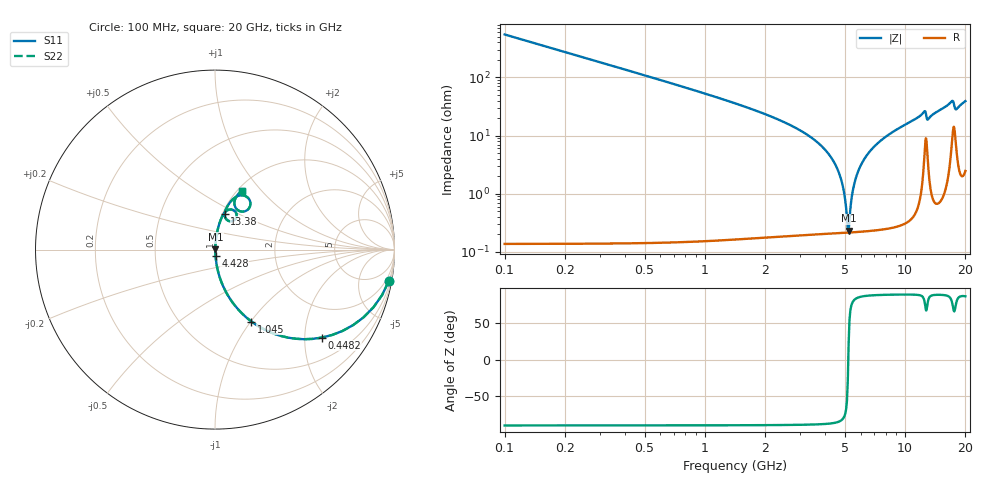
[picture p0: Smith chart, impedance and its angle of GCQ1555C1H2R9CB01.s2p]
!Murata Part Number: GCQ1555C1H2R9CB01
!These Parameters are Measured in Series Mode Connection
!Data Generated on Jan 08, 2026
!  o--ll--o
!Port1  Port2
!  o------o
!Operation Temp=25[degC], DC Bias Voltage=0[V]
!Freq. Start=100[MHz] Stop=20[GHz] 401[Steps]
# Hz S RI R 50
!Freq.(Hz) S11(Real) S11(Imag) S21(Real) S21(Imag) S12(Real) S12(Imag) S22(Real) S22(Imag)
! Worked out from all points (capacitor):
!   401 points, 100 MHz to 20 GHz, reference 50 ohm
!   read as one part in series: C = 2.9 pF near 199.5 MHz
!   lowest |Z| = 232 mohm at 5.224 GHz (marker M1)
!   series resonance near 5.203 GHz, so ESL is about 320 pH
!   S11 on the Smith chart (normalised r, x): 100 MHz: 1, -11; 448.2 MHz: 1.00, -2.43; 1.045 GHz: 1.00, -1.01; 4.428 GHz: 1.00, -0.07; 13.38 GHz: 1.02, +0.42; 20 GHz: 1.05, +0.78
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1e8  0.9678 -0.1764  0.0322 0.1764  0.0322 0.1764  0.9678 -0.1764
4.4825e8  0.5961 -0.4901  0.4039 0.4901  0.4039 0.4901  0.5961 -0.4901
1.04525e9  0.2031 -0.4008  0.7969 0.4008  0.7969 0.4008  0.2031 -0.4008
1.84125e9  0.065 -0.2433  0.935 0.2433  0.935 0.2433  0.065 -0.2433
3.43325e9  0.01 -0.0893  0.99 0.0893  0.99 0.0893  0.01 -0.0893
4.42825e9  0.00323 -0.0341  0.9968 0.0341  0.9968 0.0341  0.00323 -0.0341
4.82625e9  0.00236 -0.0158  0.9976 0.0158  0.9976 0.0158  0.00236 -0.0158
4.9755e9  0.00221 -0.00942  0.9978 0.00942  0.9978 0.00942  0.00221 -0.00942
5.12475e9  0.00214 -0.00318  0.9979 0.00318  0.9979 0.00318  0.00214 -0.00318
5.22425e9  0.00214 0.000882  0.9979 -0.000882  0.9979 -0.000882  0.00214 0.000882
5.473e9  0.00228 0.0107  0.9977 -0.0107  0.9977 -0.0107  0.00228 0.0107
5.72175e9  0.00259 0.0201  0.9974 -0.0201  0.9974 -0.0201  0.00259 0.0201
6.1695e9  0.00355 0.0362  0.9965 -0.0362  0.9965 -0.0362  0.00355 0.0362
6.7665e9  0.00548 0.0563  0.9945 -0.0563  0.9945 -0.0563  0.00548 0.0563
1.005e10  0.0264 0.1508  0.9736 -0.1508  0.9736 -0.1508  0.0264 0.1508
1.2438e10  0.0902 0.2234  0.9098 -0.2234  0.9098 -0.2234  0.0902 0.2234
1.29355e10  0.0713 0.1621  0.9287 -0.1621  0.9287 -0.1621  0.0713 0.1621
1.338325e10  0.0538 0.1985  0.9462 -0.1985  0.9462 -0.1985  0.0538 0.1985
1.67165e10  0.135 0.3009  0.865 -0.3009  0.865 -0.3009  0.135 0.3009
1.7413e10  0.1973 0.2519  0.8027 -0.2519  0.8027 -0.2519  0.1973 0.2519
1.79105e10  0.1252 0.2215  0.8748 -0.2215  0.8748 -0.2215  0.1252 0.2215
2e10  0.1482 0.3252  0.8518 -0.3252  0.8518 -0.3252  0.1482 0.3252
